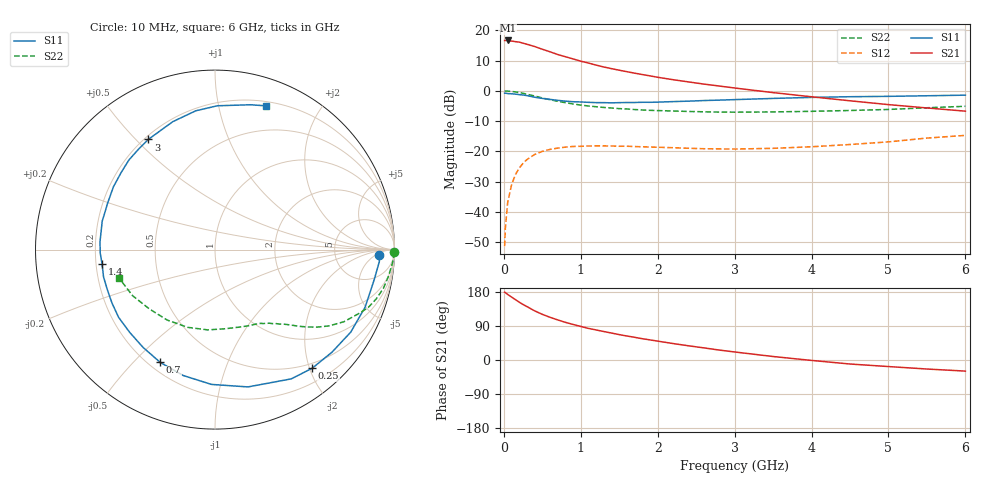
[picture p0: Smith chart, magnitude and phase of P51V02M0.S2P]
! SIEMENS Small Signal Semiconductors
! BFP183
! Si NPN RF Bipolar Junction Transistor in SOT143
! VCE = 1 V  IC = 2 mA
! Common Emitter S-Parameters:  March  1996
# GHz  S  MA  R  50
!  f  S11  S21  S12  S22
! GHz  MAG  ANG  MAG  ANG  MAG  ANG  MAG  ANG
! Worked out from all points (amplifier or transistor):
!   36 points, 10 MHz to 6 GHz, reference 50 ohm
!   highest |S21| = 16.7 dB at 50 MHz (marker M1)
!   |S21| within 3 dB of that: start of sweep to 510.9 MHz
!   unconditionally stable (mu >= 1): 2.016 GHz to end of sweep
!   at 250 MHz: K = 0.12, MSG = 19.9 dB, |S12| = -23.9 dB
!   at 1.4 GHz: K = 0.70, MSG = 12.8 dB, |S12| = -18.2 dB
!   at 6 GHz: K = 1.07, MAG = 2.4 dB, |S12| = -14.7 dB
!   S11 on the Smith chart (normalised r, x): 10 MHz: 20, -8; 250 MHz: 0.42, -2.04; 700 MHz: 0.24, -0.60; 1.4 GHz: 0.22, -0.06; 3 GHz: 0.21, +0.54; 6 GHz: 0.24, +1.39
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0.01  0.916 -1.9  6.827 179.0  0.0027 87.6  0.9975 -0.9
0.02  0.918 -4.2  6.823 177.8  0.0054 83.7  0.9971 -1.8
0.05  0.9029 -10.6  6.831 173.0  0.0143 85.6  0.9912 -4.4
0.1  0.8958 -21.0  6.684 166.1  0.0278 78.1  0.9781 -8.7
0.2  0.8668 -41.3  6.42 152.6  0.0529 66.7  0.9396 -17.0
0.25  0.8545 -50.7  6.152 146.4  0.0635 61.7  0.9127 -20.7
0.3  0.8361 -59.5  5.913 141.0  0.0731 57.1  0.8812 -23.6
0.4  0.7868 -76.5  5.424 129.7  0.0888 48.5  0.8235 -29.2
0.5  0.7514 -91.5  4.887 120.5  0.0999 41.2  0.7644 -33.8
0.6  0.7235 -104.2  4.437 112.7  0.1077 35.5  0.7142 -37.2
0.7  0.6985 -115.9  3.997 105.8  0.1132 30.6  0.6734 -39.8
0.8  0.6765 -126.3  3.677 99.4  0.1174 26.3  0.6382 -42.1
0.9  0.6622 -135.9  3.383 93.8  0.1204 22.9  0.6083 -44.0
1.1  0.6466 -152.6  2.887 83.4  0.1228 17.3  0.5628 -47.5
1.4  0.6343 -172.6  2.334 71.1  0.1227 11.1  0.5211 -52.3
1.8  0.6481 165.8  1.865 56.2  0.1191 7.6  0.483 -58.3
2.2  0.6654 148.3  1.532 43.4  0.1148 5.5  0.465 -65.5
3  0.7175 121.2  1.117 21.2  0.1091 8.1  0.4445 -82.8
3.5  0.7505 108.3  0.937 9.2  0.1122 11.8  0.4491 -95.1
4.5  0.8014 89.1  0.686 -10.6  0.1298 17.2  0.4744 -124.2
5.5  0.831 76.2  0.522 -23.8  0.1658 17.6  0.5264 -150.9
6  0.85 70.4  0.462 -29.3  0.1837 14.4  0.5562 -163.2
